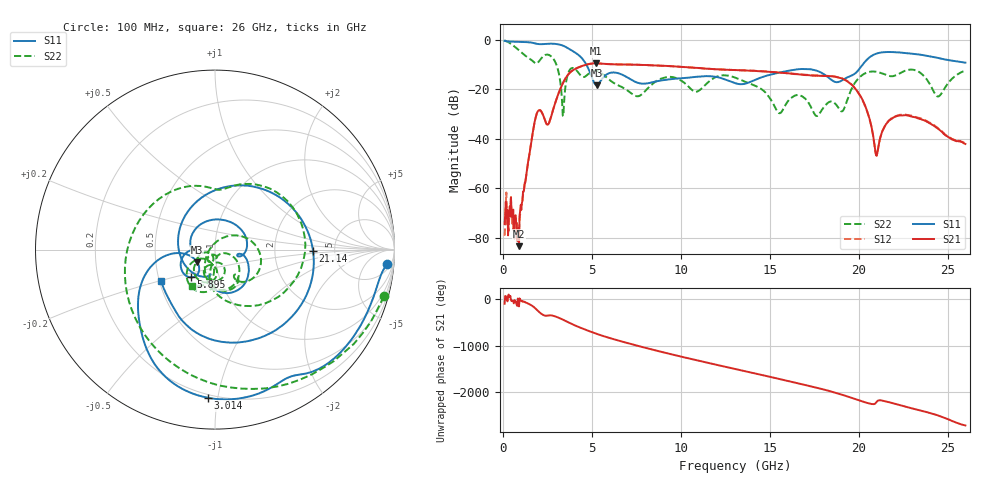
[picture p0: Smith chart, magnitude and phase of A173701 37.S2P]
!  2-Port S-parameters saved by WinCal
! VAR MeasName=S-Parameters (CALIBRATED_DATA) read from VNA (N5245A)
! VAR MeasDate=2017-6-7 10:30:53
! VAR NAME=A173701 37
! VAR FILENAME=A173701 37.S2P
! VAR DATE=2017-6-7 10:30:53
! VAR PHYS_PORTS=1,2
# Hz S DB R 50
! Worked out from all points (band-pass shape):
!   801 points, 100 MHz to 26 GHz, reference 50 ohm
!   highest |S21| = -9.48 dB at 5.248 GHz (marker M1); lowest = -83.5 dB at 909.4 MHz (marker M2)
!   |S21| within 3 dB of the highest: 3.897 GHz to 14.16 GHz (10.26 GHz wide, 114 % of centre)
!   lowest |S11| = -18.3 dB at 5.28 GHz (marker M3), VSWR 1.28, Z = 40.6 - j5.87 ohm
!   |S11| at or under -10 dB: 4.694 GHz to 20.23 GHz (15.53 GHz wide, 125 % of centre)
!   |S22| runs from -30.8 to -0.2 dB; largest |S21 - S12| = 0.0044
!   S11 on the Smith chart (normalised r, x): 100 MHz: 9, -19; 3.014 GHz: 0.18, -0.94; 5.895 GHz: 0.73, -0.24; 21.14 GHz: 3.41, -0.06; 26 GHz: 0.51, -0.21
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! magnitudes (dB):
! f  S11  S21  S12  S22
! 100 MHz  -0.3  -74.5  -79.2  -0.2
! 909.4 MHz  -0.8  -83.5  -77.7  -4.2
! 1.881 GHz  -1.5  -30.4  -30.4  -9.5
! 2.561 GHz  -1.5  -34.1  -34.1  -6.0
! 3.014 GHz  -1.7  -24.0  -23.9  -10.1
! 3.37 GHz  -2.3  -17.6  -17.5  -30.6
! 3.791 GHz  -3.9  -13.1  -13.0  -11.8
! 4.438 GHz  -7.4  -10.6  -10.6  -14.8
! 5.248 GHz  -18.3  -9.5  -9.5  -12.4
! 5.28 GHz  -18.3  -9.5  -9.5  -12.5
! 5.895 GHz  -13.7  -9.8  -9.8  -15.6
! 7.546 GHz  -17.3  -10.0  -10.0  -22.8
! 8.744 GHz  -16.6  -10.4  -10.4  -16.2
! 13.05 GHz  -17.5  -12.2  -12.2  -15.2
! 15.51 GHz  -13.3  -13.2  -13.2  -29.6
! 17.39 GHz  -12.0  -14.4  -14.3  -28.2
! 19.07 GHz  -16.3  -15.6  -15.6  -28.9
! 19.69 GHz  -14.1  -18.6  -18.7  -18.6
! 21.14 GHz  -5.3  -41.9  -41.8  -13.1
! 21.69 GHz  -4.9  -32.7  -32.7  -14.5
! 24.48 GHz  -7.3  -36.0  -35.9  -22.9
! 26 GHz  -9.2  -42.1  -41.8  -12.4
